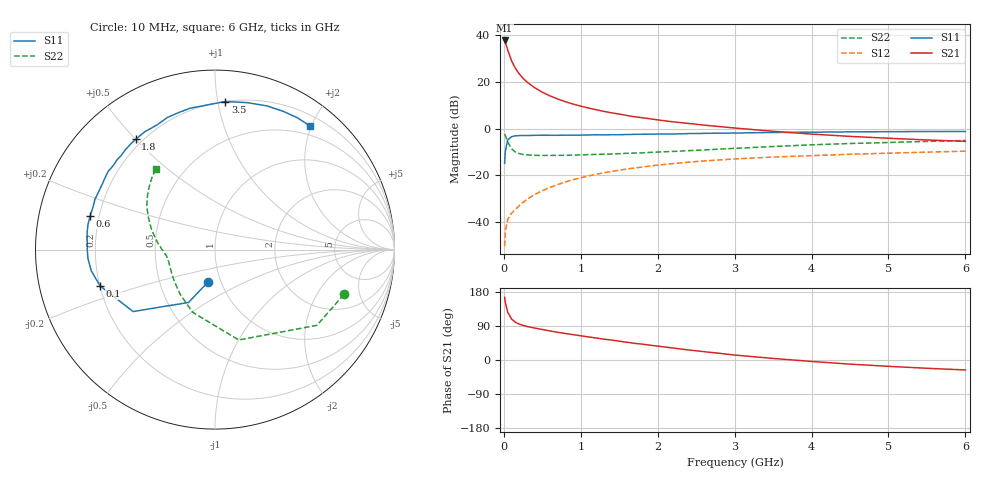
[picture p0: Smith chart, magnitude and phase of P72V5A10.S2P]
! SIEMENS Small Signal Semiconductors
! BFP196
! Si NPN RF Bipolar Junction Transistor in SOT143
! VCE = 2.5 V  IC = 100 mA
! Common Emitter S-Parameters:  May  1996
# GHz  S  MA  R  50
!  f  S11  S21  S12  S22
! GHz  MAG  ANG  MAG  ANG  MAG  ANG  MAG  ANG
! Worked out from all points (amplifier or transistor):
!   36 points, 10 MHz to 6 GHz, reference 50 ohm
!   highest |S21| = 37.6 dB at 10 MHz (marker M1)
!   |S21| within 3 dB of that: start of sweep to 40.57 MHz
!   unconditionally stable (mu >= 1): 278.3 MHz to 4.949 GHz
!   at 250 MHz: K = 0.97, MSG = 26.4 dB, |S12| = -31.4 dB
!   at 1.4 GHz: K = 1.11, MAG = 10.5 dB, |S12| = -18.3 dB
!   at 6 GHz: K = 1.00, MSG = 2.1 dB, |S12| = -9.6 dB
!   S11 on the Smith chart (normalised r, x): 10 MHz: 0.87, -0.32; 100 MHz: 0.20, -0.15; 600 MHz: 0.17, +0.13; 1.8 GHz: 0.17, +0.50; 3.5 GHz: 0.20, +1.05; 6 GHz: 0.35, +1.98
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0.01  0.1818 -101.6  75.94 165.4  0.0031 71.8  0.7605 -19.2
0.02  0.3294 -116.6  69.33 151.6  0.0064 67.4  0.7074 -36.6
0.05  0.5721 -142.9  47.85 126.2  0.0115 53.5  0.5204 -75.3
0.1  0.671 -162.4  28.05 108.2  0.0157 53.4  0.371 -109.5
0.15  0.6996 -170.3  19.37 99.9  0.0189 56.2  0.3165 -127.6
0.2  0.7092 -175.8  14.73 94.7  0.0227 59.7  0.2927 -138.5
0.25  0.7118 -179.6  11.8 91.3  0.0268 61.7  0.281 -146.3
0.3  0.7122 177.5  9.884 88.6  0.0307 64.3  0.275 -151.2
0.4  0.7189 172.4  7.469 84.3  0.0392 66.3  0.2689 -158.4
0.5  0.7212 168.7  5.977 80.5  0.0471 67.2  0.267 -162.8
0.6  0.7204 164.8  4.988 76.7  0.0557 67.4  0.2672 -165.9
0.7  0.7198 160.7  4.287 73.0  0.0639 66.8  0.2682 -168.3
0.8  0.7252 157.3  3.75 70.0  0.0728 65.8  0.2702 -170.1
1.1  0.7313 147.1  2.747 60.9  0.098 62.6  0.278 -174.6
1.4  0.7402 137.7  2.167 52.7  0.1214 58.2  0.2873 -178.0
1.8  0.7571 125.7  1.705 41.8  0.1517 52.0  0.3038 177.4
2.2  0.7656 115.1  1.394 31.6  0.1793 45.8  0.3254 172.2
3  0.8027 95.8  1.029 13.1  0.2251 33.4  0.3782 160.8
3.5  0.8271 86.0  0.876 4.1  0.2468 26.3  0.4144 153.8
4.5  0.8512 70.2  0.682 -10.9  0.2835 14.1  0.4803 141.7
5.5  0.8663 57.9  0.572 -21.8  0.3146 3.2  0.5324 131.4
6  0.8683 52.5  0.535 -26.3  0.3296 -2.6  0.5574 126.4
